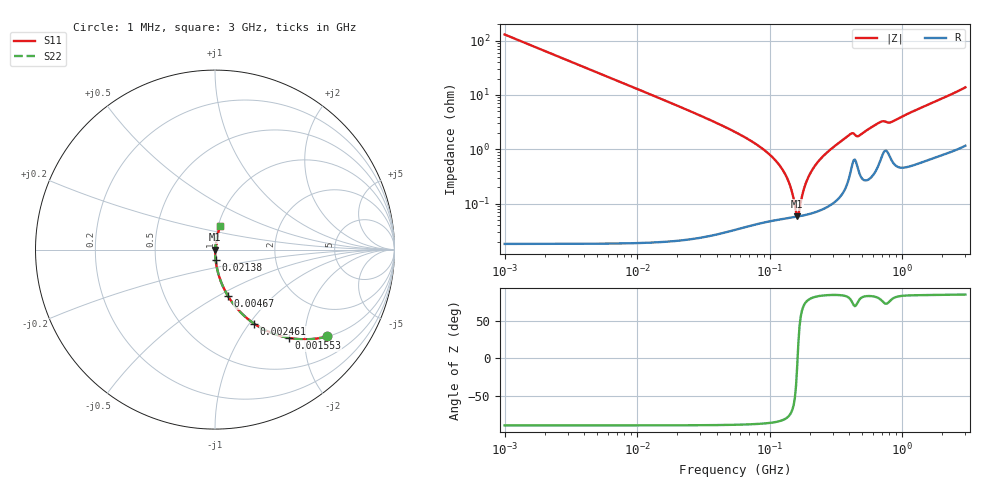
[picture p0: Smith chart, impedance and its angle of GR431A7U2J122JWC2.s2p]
!Murata Part Number: GR431A7U2J122JWC2
!These Parameters are Measured in Series Mode Connection
!Data Generated on Jun 10, 2025
!  o--ll--o
!Port1  Port2
!  o------o
!Operation Temp=25[degC], DC Bias Voltage=0[V]
!Freq. Start=1000[kHz] Stop=3[GHz] 401[Steps]
# Hz S RI R 50
!Freq.(Hz) S11(Real) S11(Imag) S21(Real) S21(Imag) S12(Real) S12(Imag) S22(Real) S22(Imag)
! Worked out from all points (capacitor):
!   401 points, 1 MHz to 3 GHz, reference 50 ohm
!   read as one part in series: C = 1.23 nF near 1.041 MHz
!   lowest |Z| = 58.6 mohm at 161.4 MHz (marker M1)
!   series resonance near 162.5 MHz, so ESL is about 780 pH
!   S11 on the Smith chart (normalised r, x): 1 MHz: 1.00, -2.59; 1.553 MHz: 1.00, -1.67; 2.461 MHz: 1.00, -1.05; 4.67 MHz: 1.00, -0.55; 21.38 MHz: 1.00, -0.12; 3 GHz: 1.02, +0.28
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1000000  0.6268 -0.4836  0.3732 0.4836  0.3732 0.4836  0.6268 -0.4836
1553251  0.4104 -0.4918  0.5896 0.4918  0.5896 0.4918  0.4104 -0.4918
2461366  0.2171 -0.4121  0.7829 0.4121  0.7829 0.4121  0.2171 -0.4121
3823119  0.1031 -0.3038  0.8969 0.3038  0.8969 0.3038  0.1031 -0.3038
4670311  0.0715 -0.2574  0.9285 0.2574  0.9285 0.2574  0.0715 -0.2574
1.461624e7  0.00786 -0.0872  0.9921 0.0872  0.9921 0.0872  0.00786 -0.0872
2.137957e7  0.00373 -0.0593  0.9963 0.0593  0.9963 0.0593  0.00373 -0.0593
5.477226e7  0.000762 -0.0208  0.9992 0.0208  0.9992 0.0208  0.000762 -0.0208
8.679508e7  0.00055 -0.0106  0.9994 0.0106  0.9994 0.0106  0.00055 -0.0106
1.171891e8  0.000535 -0.00526  0.9995 0.00526  0.9995 0.00526  0.000535 -0.00526
1.375402e8  0.000547 -0.00265  0.9995 0.00265  0.9995 0.00265  0.000547 -0.00265
1.614254e8  0.000576 -0.000105  0.9994 0.000105  0.9994 0.000105  0.000576 -0.000105
1.680187e8  0.000587 0.000532  0.9994 -0.000532  0.9994 -0.000532  0.000587 0.000532
1.784169e8  0.000606 0.00149  0.9994 -0.00149  0.9994 -0.00149  0.000606 0.00149
1.894586e8  0.00063 0.00246  0.9994 -0.00246  0.9994 -0.00246  0.00063 0.00246
2.094008e8  0.000683 0.00411  0.9993 -0.00411  0.9993 -0.00411  0.000683 0.00411
2.662515e8  0.000911 0.00834  0.9991 -0.00834  0.9991 -0.00834  0.000911 0.00834
4.0536e8  0.00391 0.0185  0.9961 -0.0185  0.9961 -0.0185  0.00391 0.0185
4.66327e8  0.00446 0.0168  0.9955 -0.0168  0.9955 -0.0168  0.00446 0.0168
6.821091e8  0.00697 0.0306  0.993 -0.0306  0.993 -0.0306  0.00697 0.0306
8.005644e8  0.00844 0.0296  0.9916 -0.0296  0.9916 -0.0296  0.00844 0.0296
3e9  0.0294 0.132  0.9706 -0.132  0.9706 -0.132  0.0294 0.132
